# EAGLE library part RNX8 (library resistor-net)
RESISTOR NETWORK
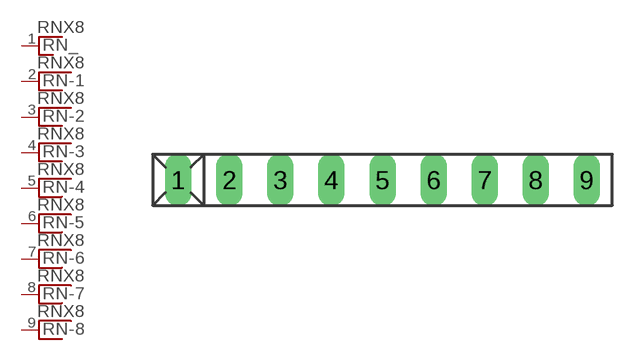
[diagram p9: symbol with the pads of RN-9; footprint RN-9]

Designator prefix RN; gates _=RN_1 -1=RNX -2=RNX -3=RNX -4=RNX -5=RNX -6=RNX -7=RNX -8=RNX

## RNX8 (OC_FARNELL: unknown; OC_NEWARK: unknown)  [RN-9]
1  _:1  pas
2  -1:1  pas
3  -2:1  pas
4  -3:1  pas
5  -4:1  pas
6  -5:1  pas
7  -6:1  pas
8  -7:1  pas
9  -8:1  pas

## Footprint RN-9 (pad centres in mm)
RESISTOR NETWORK
drill 0.813 long: 1 -10.16,0; 2 -7.62,0; 3 -5.08,0; 4 -2.54,0; 5 0,0; 6 2.54,0; 7 5.08,0; 8 7.62,0; 9 10.16,0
